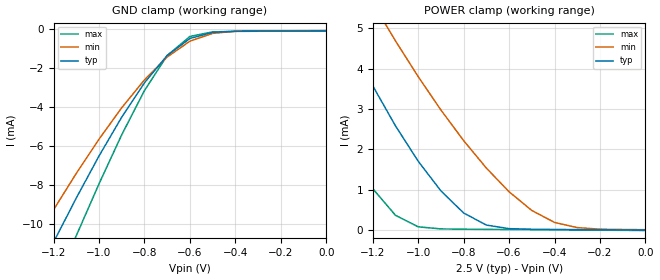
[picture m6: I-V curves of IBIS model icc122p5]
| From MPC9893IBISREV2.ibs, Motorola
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|This model is an Input with a 25,000 ohm Pull_up at 2.5V
[Model]   icc122p5
Model_type   Input
Polarity   Non-Inverting
Vmeas=1.25
Vinl=0.7
Vinh=1.7
| Variable   typ   min   max
C_comp   5p   5p   5p
[Temperature Range]   27.00   100.00   -45.00
[Power Clamp Reference]   2.50V   2.25V   2.75V
[Gnd Clamp Reference]   0.000V   0.000V   0.000V
[Voltage Range]   2.50V   2.25V   2.75V
[Pulldown Reference]   0.000V   0.000V   0.000V
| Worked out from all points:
|   GND clamp passes 1 mA (typ) near -0.66 V on its own axis
|   POWER clamp passes 1 mA (typ) near -0.90 V on its own axis
[GND_clamp]
| voltage   I(typ)   I(min)   I(max)
-2.5V     -43.6mA    -37.69mA   -50.1mA
-1.3V     -13.31mA   -11.24mA   -16.16mA
-1.2V     -10.96mA   -9.292mA   -13.37mA
-1.1V     -8.69mA    -7.426mA   -10.63mA
-1V       -6.532mA   -5.668mA   -7.963mA
-900mV    -4.534mA   -4.051mA   -5.441mA
-800mV    -2.77mA    -2.62mA    -3.17mA
-700mV    -1.364mA   -1.445mA   -1.369mA
-600mV    -492.2uA   -630.4uA   -388.8uA
-500mV    -177.4uA   -229uA     -153.4uA
-400mV    -120.2uA   -121.1uA   -125.9uA
1.08fV    -99.01uA   -89.11uA   -108.9uA
[POWER_clamp]
| voltage   I(typ)  I(min)  I(max)
-2.5V     21.34mA    20.61mA    21.16mA
-1.6V     8.35mA     9.799mA    5.904mA
-1.5V     7.062mA    8.704mA    4.467mA
-1.3V     4.663mA    6.615mA    1.984mA
-1.2V     3.577mA    5.629mA    1.028mA
-1.1V     2.585mA    4.69mA     367.6uA
-1V       1.708mA    3.804mA    80.99uA
-800mV    424.6uA    2.218mA    21.92uA
-700mV    124.2uA    1.537mA    17.82uA
-500mV    20.84uA    486.4uA    9.901uA
-400mV    15.91uA    189.6uA    5.941uA
1.08fV    26.02pA    9.938uA    -9.901uA
